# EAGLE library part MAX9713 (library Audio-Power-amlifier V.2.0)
The MAX9713 mono/stereo Class D audio power amplifiers provide Class AB amplifier performance with Class D efficiency, conserving board space and eliminating the need for a bulky heatsink. Using a Class D architecture, these devices deliver up to 6W while offering greater than 85% efficiency. Proprietary and protected modulation and switching schemes render the traditional Class D output filter unnecessary.
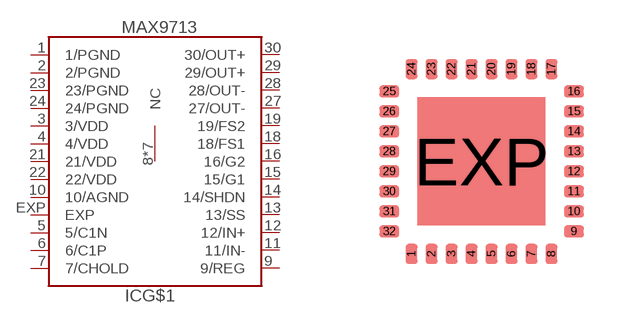
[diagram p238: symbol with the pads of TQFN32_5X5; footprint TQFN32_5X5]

Designator prefix IC; gates G$1=MAX9713 G$2=NC

## MAX9713  [TQFN32_5X5]
1  G$1:1/PGND  pwr
2  G$1:2/PGND  pwr
3  G$1:3/VDD  pwr
4  G$1:4/VDD  pwr
5  G$1:5/C1N
6  G$1:6/C1P
7  G$1:7/CHOLD
8  G$2:NC  nc
9  G$1:9/REG  out
10  G$1:10/AGND  pwr
11  G$1:11/IN-  in
12  G$1:12/IN+  in
13  G$1:13/SS
14  G$1:14/SHDN
15  G$1:15/G1  in
16  G$1:16/G2  in
17  G$2:NC  nc
18  G$1:18/FS1  in
19  G$1:19/FS2  in
20  G$2:NC  nc
21  G$1:21/VDD  pwr
22  G$1:22/VDD  pwr
23  G$1:23/PGND  pwr
24  G$1:24/PGND  pwr
25  G$2:NC  nc
26  G$2:NC  nc
27  G$1:27/OUT-  out
28  G$1:28/OUT-  out
29  G$1:29/OUT+  out
30  G$1:30/OUT+  out
31  G$2:NC  nc
32  G$2:NC  nc
EXP  G$1:EXP  pwr

## Footprint TQFN32_5X5 (pad centres in mm)
TQFN32-5x5x0,8mm. Source: www.maxim-ic.com/packages
smd 0.3 x 0.5: 1 -1.75,-2.31; 2 -1.25,-2.31; 3 -0.75,-2.31; 4 -0.25,-2.31; 5 0.25,-2.31; 6 0.75,-2.31; 7 1.25,-2.31; 8 1.75,-2.31; 17 1.75,2.31; 18 1.25,2.31; 19 0.75,2.31; 20 0.25,2.31; 21 -0.25,2.31; 22 -0.75,2.31; 23 -1.25,2.31; 24 -1.75,2.31
smd 0.5 x 0.3: 9 2.31,-1.75; 10 2.31,-1.25; 11 2.31,-0.75; 12 2.31,-0.25; 13 2.31,0.25; 14 2.31,0.75; 15 2.31,1.25; 16 2.31,1.75; 25 -2.31,1.75; 26 -2.31,1.25; 27 -2.31,0.75; 28 -2.31,0.25; 29 -2.31,-0.25; 30 -2.31,-0.75; 31 -2.31,-1.25; 32 -2.31,-1.75
smd 3.2 x 3.2: EXP 0,0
